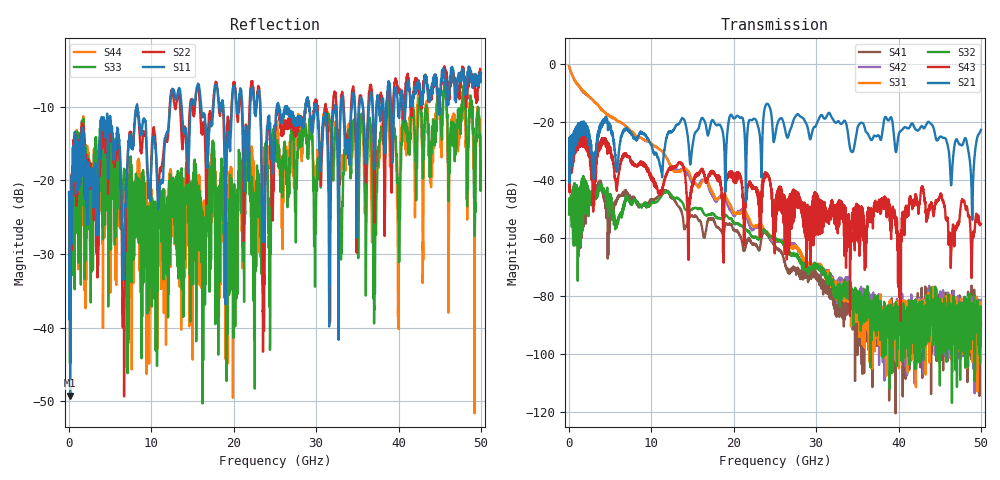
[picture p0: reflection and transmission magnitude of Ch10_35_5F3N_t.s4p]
!Agilent Technologies,N5247A,US51170199,A.09.90.13
!Agilent N5247A: A.09.90.13
!Date: Wednesday, December 16, 2015 12:31:24
!Correction: S11(Full 4 Port(1,2,3,4))
!S12(Full 4 Port(1,2,3,4))
!S13(Full 4 Port(1,2,3,4))
!S14(Full 4 Port(1,2,3,4))
!S21(Full 4 Port(1,2,3,4))
!S22(Full 4 Port(1,2,3,4))
!S23(Full 4 Port(1,2,3,4))
!S24(Full 4 Port(1,2,3,4))
!S31(Full 4 Port(1,2,3,4))
!S32(Full 4 Port(1,2,3,4))
!S33(Full 4 Port(1,2,3,4))
!S34(Full 4 Port(1,2,3,4))
!S41(Full 4 Port(1,2,3,4))
!S42(Full 4 Port(1,2,3,4))
!S43(Full 4 Port(1,2,3,4))
!S44(Full 4 Port(1,2,3,4))
!S4P File: Measurements: <S11,S12,S13,S14>,
!<S21,S22,S23,S24>,
!<S31,S32,S33,S34>,
!<S41,S42,S43,S44>:
# Hz S  dB  R 50
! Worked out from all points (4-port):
!   3201 points, 10 MHz to 50 GHz, reference 50 ohm
!   strongest paths, dB at 10 MHz, 12.51 GHz, 25 GHz, 37.5 GHz, 50 GHz:
!     S21: -32.5, -23.4, -25.2, -24.7, -22.8
!     S43: -32.8, -35.5, -48.9, -48.5, -55.2
!     S32: -52.0, -45.7, -60.4, -90.5, -88.7
!     S31: -0.9, -36.2, -60.9, -82.0, -93.0
!     S42: -0.9, -35.8, -61.0, -83.9, -81.5
!     S41: -52.0, -46.3, -62.9, -83.2, -90.3
!   lowest |S11| = -49.2 dB at 135 MHz (marker M1), VSWR 1.01, Z = 49.8 + j0.307 ohm
!   |S11| at or under -10 dB: start of sweep to 8.229 GHz; 8.28 GHz to 12.26 GHz (3.985 GHz wide, 38.8 % of centre); 26.46 GHz to 28.7 GHz (2.239 GHz wide, 8.12 % of centre)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
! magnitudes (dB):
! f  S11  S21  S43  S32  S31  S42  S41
! 10 MHz  -21.6  -32.5  -32.8  -52.0  -0.9  -0.9  -52.0
! 135 MHz  -49.2  -32.8  -34.0  -46.9  -2.1  -2.1  -47.0
! 11.84 GHz  -13.6  -25.7  -37.9  -44.3  -32.5  -32.3  -43.9
! 23.63 GHz  -23.8  -17.7  -40.6  -57.2  -57.0  -57.1  -58.4
! 32.41 GHz  -11.2  -20.4  -49.6  -78.7  -80.9  -76.4  -86.8
! 48.92 GHz  -6.1  -50.8  -66.6  -88.5  -92.3  -92.9  -99.7
! 50 GHz  -5.6  -22.8  -55.2  -88.7  -93.0  -81.5  -90.3
